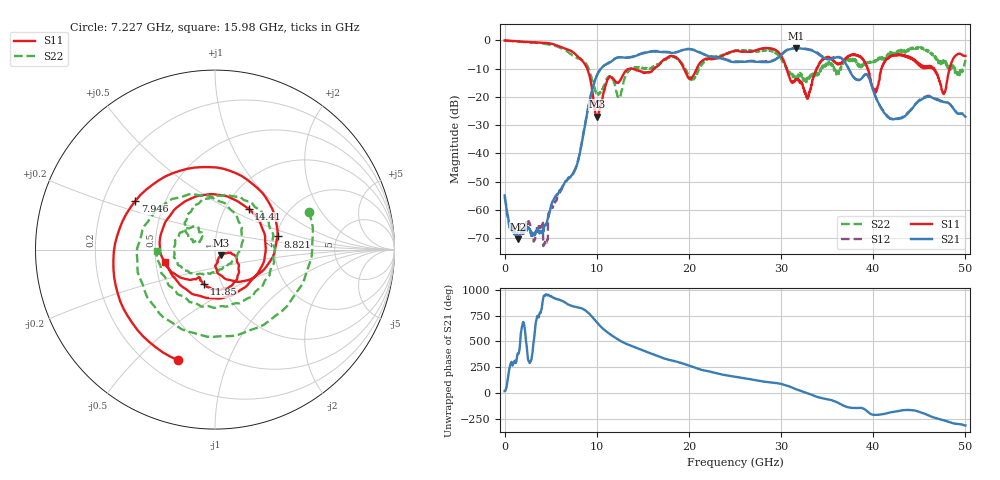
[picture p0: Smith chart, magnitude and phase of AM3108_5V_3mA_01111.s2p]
# Hz S DB R 50.0
!freq dBS11 angS11 dBS21 angS21 dBS12 angS12 dBS22 angS22
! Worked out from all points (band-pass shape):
!   1601 points, 10 MHz to 50 GHz, reference 50 ohm
!   highest |S21| = -2.77 dB at 31.66 GHz (marker M1); lowest = -70.5 dB at 1.447 GHz (marker M2)
!   |S21| within 3 dB of the highest: 13.97 GHz to 22.48 GHz (8.503 GHz wide, 46.7 % of centre); 29.82 GHz to 34.45 GHz (4.627 GHz wide, 14.4 % of centre)
!   lowest |S11| = -26.9 dB at 10.04 GHz (marker M3), VSWR 1.09, Z = 53.3 - j3.32 ohm
!   |S11| at or under -10 dB: 8.968 GHz to 13.59 GHz (4.627 GHz wide, 41 % of centre); 13.85 GHz to 16.23 GHz (2.377 GHz wide, 15.8 % of centre); 30.62 GHz to 33.85 GHz (3.229 GHz wide, 10 % of centre)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
!   |S22| runs from -20.5 to 0.0 dB; largest |S21 - S12| = 0.026
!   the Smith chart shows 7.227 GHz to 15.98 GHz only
!   S11 on the Smith chart (normalised r, x): 7.227 GHz: 0.32, -0.67; 7.946 GHz: 0.34, +0.25; 8.821 GHz: 2.03, +0.34; 11.85 GHz: 0.83, -0.33; 14.41 GHz: 1.28, +0.64; 15.98 GHz: 0.56, -0.09
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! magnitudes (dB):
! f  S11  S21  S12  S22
! 10 MHz  0.0  -54.9  -55.4  0.0
! 1.447 GHz  -0.3  -70.5  -68.3  -0.4
! 4.447 GHz  -0.9  -65.4  -71.6  -1.2
! 7.227 GHz  -3.7  -47.9  -48.3  -5.0
! 7.946 GHz  -5.7  -43.2  -42.8  -6.3
! 8.352 GHz  -6.9  -36.9  -36.6  -6.7
! 8.821 GHz  -9.0  -28.3  -28.2  -8.0
! 10.04 GHz  -26.9  -12.2  -12.2  -18.8
! 11.85 GHz  -13.9  -6.8  -6.6  -14.6
! 14.41 GHz  -10.6  -5.2  -5.1  -9.7
! 15.98 GHz  -10.9  -3.9  -3.8  -9.8
! 16.69 GHz  -8.8  -4.0  -3.8  -8.6
! 20.41 GHz  -12.7  -3.3  -3.2  -14.0
! 25 GHz  -3.7  -7.6  -7.4  -3.8
! 29.29 GHz  -3.1  -7.0  -6.8  -4.0
! 31.66 GHz  -13.9  -2.8  -2.6  -13.6
! 33.35 GHz  -15.5  -3.6  -3.4  -12.7
! 38 GHz  -4.9  -13.6  -13.4  -6.6
! 40.22 GHz  -18.6  -19.7  -19.6  -7.6
! 41.69 GHz  -6.0  -27.3  -27.2  -5.2
! 47.66 GHz  -19.0  -21.8  -21.6  -7.7
! 50 GHz  -5.5  -27.0  -26.7  -6.9
